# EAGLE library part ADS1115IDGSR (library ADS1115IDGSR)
16-Bit 860SPS 4-Ch Delta-Sigma ADC With PGA, Oscillator, Vref, Comparator, and I2C Source: Datasheet
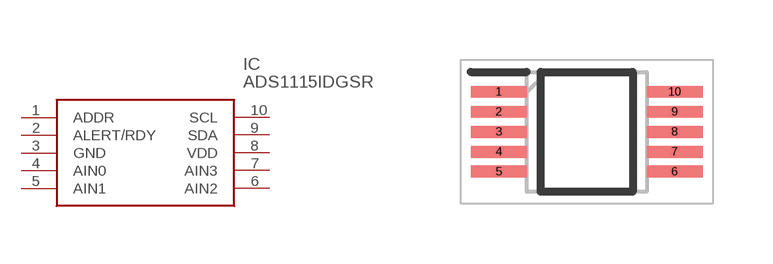
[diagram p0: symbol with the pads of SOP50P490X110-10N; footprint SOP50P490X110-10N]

Designator prefix IC

## ADS1115IDGSR (Arrow_Part_Number: ADS1115IDGSR; Arrow_Price-Stock: https://www.arrow.com/en/products/ads1115idgsr/texas-instruments?region=nac; Description: 16-Bit 860SPS 4-Ch Delta-Sigma ADC With PGA, Oscillator, Vref, Comparator, and I2C; Height: 1.1mm; Manufacturer_Name: Texas Instruments; Manufacturer_Part_Number: ADS1115IDGSR; Mouser_Part_Number: 595-ADS1115IDGSR; Mouser_Price-Stock: https://www.mouser.co.uk/ProductDetail/Texas-Instruments/ADS1115IDGSR?qs=IK5e5L0zOXjKCJoVMhYO%2FQ%3D%3D)  [SOP50P490X110-10N]
1  ADDR
2  ALERT/RDY
3  GND
4  AIN0
5  AIN1
6  AIN2
7  AIN3
8  VDD
9  SDA
10  SCL

## Footprint SOP50P490X110-10N (pad centres in mm)
DGS0010A
smd 1.4 x 0.3: 1 -2.2,1; 2 -2.2,0.5; 3 -2.2,0; 4 -2.2,-0.5; 5 -2.2,-1; 6 2.2,-1; 7 2.2,-0.5; 8 2.2,0; 9 2.2,0.5; 10 2.2,1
